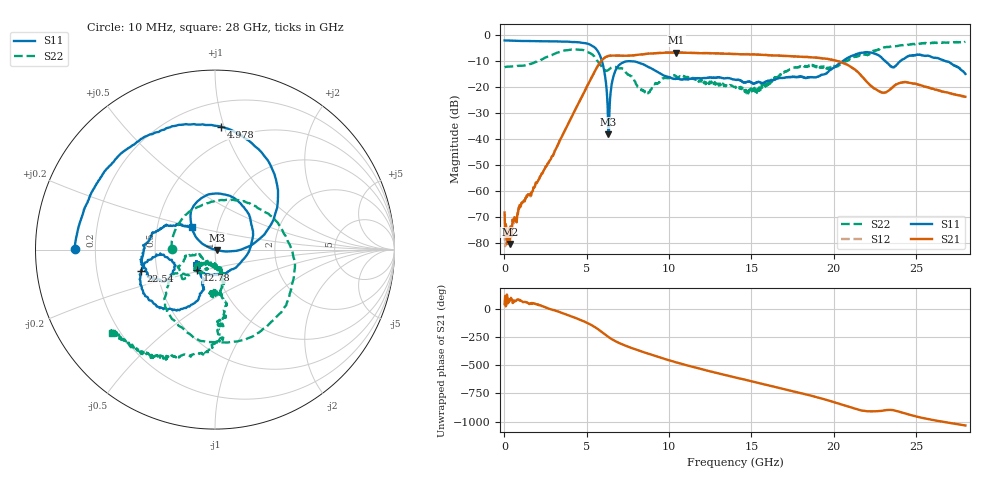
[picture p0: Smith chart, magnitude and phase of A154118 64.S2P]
!  2-Port S-parameters saved by WinCal
! VAR MeasName=S-Parameters (CALIBRATED_DATA) read from VNA (N5230A)
! VAR MeasDate=2015-9-10 14:40:04
! VAR NAME=A154118 64
! VAR FILENAME=A154118 64.S2P
! VAR DATE=2015-9-10 14:40:04
! VAR PHYS_PORTS=1,2
# Hz S DB R 50
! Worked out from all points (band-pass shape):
!   801 points, 10 MHz to 28 GHz, reference 50 ohm
!   highest |S21| = -6.79 dB at 10.44 GHz (marker M1); lowest = -80.4 dB at 324.9 MHz (marker M2)
!   |S21| within 3 dB of the highest: 5.917 GHz to 20.06 GHz (14.14 GHz wide, 109 % of centre)
!   lowest |S11| = -38.3 dB at 6.308 GHz (marker M3), VSWR 1.02, Z = 51.2 - j0.259 ohm
!   |S11| at or under -10 dB: 5.919 GHz to 20.57 GHz (14.65 GHz wide, 111 % of centre); 23.12 GHz to 24.06 GHz (940.5 MHz wide, 3.99 % of centre); 26.74 GHz to end of sweep
!   |S22| runs from -22.5 to -2.7 dB; largest |S21 - S12| = 0.0085
!   S11 on the Smith chart (normalised r, x): 10 MHz: 0.12, +0.00; 4.978 GHz: 0.38, +0.98; 12.78 GHz: 0.80, -0.19; 22.54 GHz: 0.41, -0.12; 28 GHz: 0.75, +0.19
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1e7  -2.15 179.7  -68.21 40.2  -75.69 -42.3  -12.49 179.7
3.248875e8  -2.20 175.2  -80.36 82.8  -78.62 56.1  -12.20 160.0
1.934312e9  -2.42 154.6  -56.70 37.9  -56.86 36.2  -10.31 63.4
3.158875e9  -2.51 135.5  -43.33 -20.9  -43.31 -21.0  -6.95 -8.8
4.698325e9  -3.05 98.4  -23.81 -105.0  -23.83 -105.4  -5.78 -97.0
4.978225e9  -3.27 87.1  -20.26 -122.4  -20.26 -122.1  -6.39 -110.4
5.852912e9  -8.70 27.2  -10.28 160.5  -10.28 160.5  -11.71 -149.5
6.30775e9  -38.26 -12.0  -8.11 110.3  -8.09 110.2  -13.51 -134.5
6.657625e9  -15.19 137.3  -7.94 78.7  -7.94 78.6  -12.23 -138.1
7.077475e9  -11.06 112.1  -8.05 48.9  -8.04 48.6  -12.89 -154.3
8.581938e9  -11.82 39.8  -7.32 -31.1  -7.30 -31.1  -21.81 -130.4
9.351662e9  -14.40 -2.6  -6.99 -67.8  -6.95 -67.9  -18.49 -115.6
1.043628e10  -16.75 -61.2  -6.79 -115.3  -6.77 -115.6  -15.87 -125.4
1.278044e10  -16.40 -130.4  -7.08 155.4  -7.04 154.8  -18.16 -131.4
1.4005e10  -17.20 -145.5  -7.36 112.0  -7.34 111.6  -20.05 -129.1
1.662906e10  -16.76 -130.7  -7.96 21.7  -7.93 20.8  -15.95 -71.5
1.869332e10  -16.22 -124.8  -8.62 -52.1  -8.67 -52.7  -11.51 -92.7
2.07226e10  -9.31 -113.9  -11.19 -139.1  -11.19 -139.9  -10.20 -77.6
2.254195e10  -7.37 -163.7  -20.81 172.3  -20.89 171.2  -6.03 -84.6
2.334666e10  -11.42 -170.9  -21.39 -175.6  -21.49 -176.7  -4.66 -99.0
2.5201e10  -7.71 -171.7  -19.22 119.8  -19.27 119.1  -3.39 -118.1
2.8e10  -15.01 136.1  -23.78 46.8  -23.83 46.0  -2.65 -141.0
